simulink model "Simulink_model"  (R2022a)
settings: Solver=VariableStepAuto  StartTime=0.0  StopTime=10.0  RelTol=1e-3
undefined symbols (not defined in the file): Ion, Lithium, sigbuilder_block
libraries: spsMeanLib x15, spsSeriesRLCBranchLib x5, spsIGBTDiodeLib x4, slpidlib x3, spsBatteryLib x2, spsPWMGeneratorDCDCLib x2, spsFirstOrderFilterLib x1, spsCurrentMeasurementLib x1, spsSeriesRLCLoadLib x1, spsVoltageMeasurementLib x1, spspowerguiLib x1

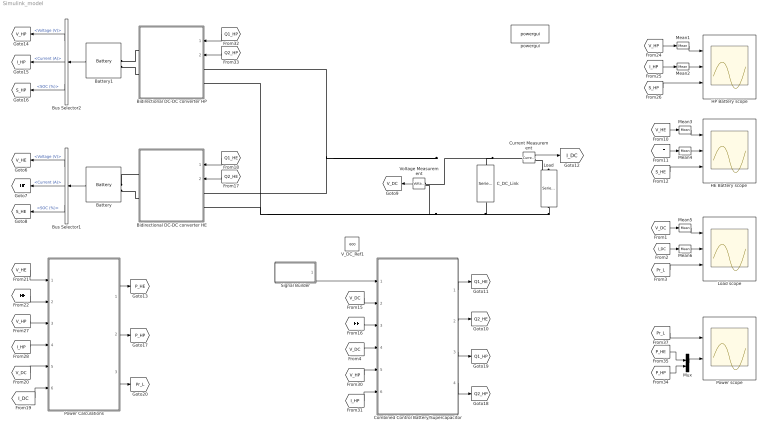
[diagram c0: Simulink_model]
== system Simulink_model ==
  Battery : spsBatteryLib/Battery  BatType=Lithium-Ion  ShowTempParam=off  ThermalPreset=no  ShowAgeParam=off  NomV=300  NomQ=120  SOC=50  Batt_Tr=0.1  PresetModel=on  MaxQ=120  MinV=225  FullV=349.1961  Dis_rate=52.1739  R=0.025  Normal_OP=108.5217  expZone="[324.1158      5.895652]"  current=[6.5 13 32.5]  Units=Time  Tci=20  NomT=20  T2=-30  MaxQ2=4.8  FullV2=7.1  Normal_OP2=5.655  expZone2="[6.58           1]"  Rca=0.6  ti=2000  Dp=0  Neq0=0  Tsim=1e6  Ta1=25  Qeol=5.4*0.9  Reol=0.013333*1.2  Char_age=[2.3478, 3]  Dis_age=[2.3478, 10]  N1=1500  N2=10500  N3=1000  N4=1400  Ta2=45  N5=950
  Battery1 : spsBatteryLib/Battery  BatType=Lithium-Ion  ShowTempParam=off  ThermalPreset=no  ShowAgeParam=off  NomV=100  NomQ=50  SOC=50  Batt_Tr=0.1  PresetModel=on  MaxQ=50  MinV=75  FullV=116.3987  Dis_rate=21.7391  R=0.02  Normal_OP=45.2174  expZone="[108.0386      2.456522]"  current=[6.5 13 32.5]  Units=Time  Tci=20  NomT=20  T2=-30  MaxQ2=4.8  FullV2=7.1  Normal_OP2=5.655  expZone2="[6.58           1]"  Rca=0.6  ti=2000  Dp=0  Neq0=0  Tsim=1e6  Ta1=25  Qeol=5.4*0.9  Reol=0.013333*1.2  Char_age=[2.3478, 3]  Dis_age=[2.3478, 10]  N1=1500  N2=10500  N3=1000  N4=1400  Ta2=45  N5=950
  Bidirectional DC-DC converter HE : Subsystem
  Bidirectional DC-DC converter HP : Subsystem
  Bus Selector1 : BusSelector  OutputSignals=Voltage (V),Current (A),SOC (%)
  Bus Selector2 : BusSelector  OutputSignals=Voltage (V),Current (A),SOC (%)
  C_DC_Link : spsSeriesRLCBranchLib/Series RLC Branch  LConnTagsString=__new0  RConnTagsString=__new0  BranchType=C  Resistance=1  Inductance=1e-3  SetiL0=off  InitialCurrent=0  Capacitance=300e-6  Setx0=off  InitialVoltage=0  Measurements=None
  Combined Control Battery/Supercapacitor : Subsystem
  Current Measurement : spsCurrentMeasurementLib/Current Measurement  PhasorSimulation=off  OutputType=Complex  PSBequivalent=0
  "HE Battery scope " : Scope  NumInputPorts=3
  HP Battery scope : Scope  NumInputPorts=3
  Load : spsSeriesRLCLoadLib/Series RLC Load  LConnTagsString=a  RConnTagsString=__new0  NominalVoltage=50  NominalFrequency=0.00001  ActivePower=500  InductivePower=0  CapacitivePower=0  Setx0=off  InitialVoltage=0  SetiL0=off  InitialCurrent=0  Measurements=None  LoadType=constant Z
  Load scope : Scope  NumInputPorts=3
  Mean{1..6} (6 alike) : spsMeanLib/Mean  Freq=60  Vinit=0  Ts=0
  Mux : Mux  Inputs=2
  Power Calculations : Subsystem
  Power scope : Scope  NumInputPorts=2
  Signal Builder : Subsystem  Tag=STV Subsys  LoadFcn=sigbuilder_block('load');  StartFcn=sigbuilder_block('start');  StopFcn=sigbuilder_block('stop');  ClipboardFcn=sigbuilder_block('clipboard');  mask(Sigbuilder block){tuvar=[0:10]}
      mask help: Simulink:masks:SigbuilderBlock_MD
      mask init:
      | if ~strcmp(get_param(bdroot(gcbh),'SimulationStatus'),'stopped') tuvar = sigbuilder_block('maskInit'); end
  V_DC_Ref1 : Constant  Value=600
  Voltage Measurement : spsVoltageMeasurementLib/Voltage Measurement  PhasorSimulation=off  OutputType=Complex  PSBequivalent=0
  powergui : spspowerguiLib/powergui  Priority=1  SimulationMode=Discrete  SampleTime=1e-6  frequency=60  Iterations=50  frequencyindice=0  Pbase=100e6  ErrMax=1e-4  UnitsV=kV  UnitsW=MW  buscounter=0  FunctionMessages=off  echomessages=off  EnableUseOfTLC=off  CurrentSourceSwitches=off  DisableSnubberDevices=off  DisableRonSwitches=off  DisableVfSwitches=off  DisplayEquations=off  AutomaticDiscreteSolvers=off  SolverType=Tustin/Backward Euler (TBE)  Interpol=off  ExternalGateDelay=off  methode=off  Ts=100  x0status=blocks  SPID=on  SwTol=0  HookPort=off  NonlinearTolerance=1e-4  nMaxIteration=100  ContinueOnMaxIteration=off  RestoreLinks=warning  ResistiveCurrentMeasurement=off  Frange=[0:2:500]  Ylog=off  Xlog=on  ShowGrid=off  save=off  variable=ZData  structure=0  ZoomFFT=off  StartTime=0.0  cycles=1  DisplayStyle=1  fundamental=60  FreqAxis=off  MaxFrequency=1000  frequencyindicesteady=1  RmsSteady=1  display=off
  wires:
  [V_HE] -> Power Calculations/1(V_HE)
  [I_DC] -> Mean6/1
  [V_DC] -> Power Calculations/5(V_DC)
  Bus Selector2/1 -> [V_HP]  "<Voltage (V)>"
  Current Measurement/1 -> [I_DC]
  Bus Selector1/3 -> [S_HE]  "<SOC (%)>"
  [I_HP] -> Mean2/1
  Power Calculations/1(P_HE) -> [P_HE]
  Combined Control Battery/Supercapacitor/1(Q1_HE) -> [Q1_HE]
  Bus Selector2/2 -> [I_HP]  "<Current (A)>"
  [P_HE] -> Mux/1
  [V_DC] -> Combined Control Battery/Supercapacitor/4(V_DC1)
  [P_HP] -> Mux/2
  [Q2_HE] -> Bidirectional DC-DC converter HE/2(D_Q2)
  [Pr_L] -> Load scope/3
  [V_HE] -> Mean3/1
  [V_HP] -> Mean1/1
  [Q1_HE] -> Bidirectional DC-DC converter HE/1(D_Q1)
  Power Calculations/3(P_Load) -> [Pr_L]
  [I_DC] -> Power Calculations/6(I_DC)
  [I_HE] -> Mean4/1
  Combined Control Battery/Supercapacitor/2(Q2_HE) -> [Q2_HE]
  [Q2_HP] -> Bidirectional DC-DC converter HP/2(D_Q2)
  [I_HP] -> Combined Control Battery/Supercapacitor/6(I_HP)
  Bus Selector2/3 -> [S_HP]  "<SOC (%)>"
  [V_HP] -> Power Calculations/3(V_HP)
  [S_HP] -> HP Battery scope/3
  [V_DC] -> Combined Control Battery/Supercapacitor/2(V_DC)
  Battery/1 -> Bus Selector1/1
  [V_DC] -> Mean5/1
  Power Calculations/2(P_HP) -> [P_HP]
  [V_HP] -> Combined Control Battery/Supercapacitor/5("V_HP ")
  Mux/1 -> Power scope/2
  Combined Control Battery/Supercapacitor/4(Q2_HP) -> [Q2_HP]
  Bus Selector1/1 -> [V_HE]  "<Voltage (V)>"
  [I_HP] -> Power Calculations/4(I_HP)
  Combined Control Battery/Supercapacitor/3(Q1_HP) -> [Q1_HP]
  [S_HE] -> "HE Battery scope "/3
  [I_HE] -> Power Calculations/2(I_HE)
  Bus Selector1/2 -> [I_HE]  "<Current (A)>"
  [Q1_HP] -> Bidirectional DC-DC converter HP/1(D_Q1)
  Battery1/1 -> Bus Selector2/1
  [I_HE] -> Combined Control Battery/Supercapacitor/3(I_HE)
  Voltage Measurement/1 -> [V_DC]
  [Pr_L] -> Power scope/1
  Signal Builder/1(Signal 1) -> Combined Control Battery/Supercapacitor/1(VDC_ref)
  Mean1/1 -> HP Battery scope/1
  Mean2/1 -> HP Battery scope/2
  Mean3/1 -> "HE Battery scope "/1
  Mean4/1 -> "HE Battery scope "/2
  Mean5/1 -> Load scope/1
  Mean6/1 -> Load scope/2
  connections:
  Load/RConn1 -- Voltage Measurement/LConn2 -- Bidirectional DC-DC converter HE/LConn2 -- Bidirectional DC-DC converter HP/LConn2 -- C_DC_Link/RConn1
  Current Measurement/LConn1 -- Voltage Measurement/LConn1 -- Bidirectional DC-DC converter HE/LConn1 -- Bidirectional DC-DC converter HP/LConn1 -- C_DC_Link/LConn1
  Bidirectional DC-DC converter HP/RConn1 -- Battery1/LConn1
  Battery/LConn1 -- Bidirectional DC-DC converter HE/RConn1
  Current Measurement/RConn1 -- Load/LConn1
  Bidirectional DC-DC converter HE/RConn2 -- Battery/LConn2
  Bidirectional DC-DC converter HP/RConn2 -- Battery1/LConn2

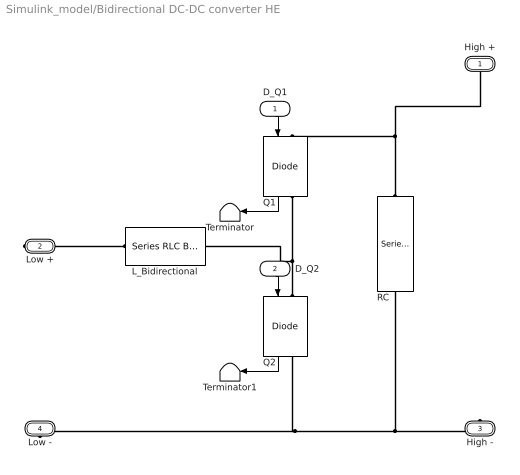
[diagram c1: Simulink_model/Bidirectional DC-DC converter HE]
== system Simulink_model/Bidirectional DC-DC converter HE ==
  D_Q1 : Inport
  D_Q2 : Inport  Port=2
  L_Bidirectional : spsSeriesRLCBranchLib/Series RLC Branch  LConnTagsString=__new0  RConnTagsString=__new0  BranchType=RL  Resistance=0.05  Inductance=0.3e-3  SetiL0=off  InitialCurrent=0  Capacitance=1e-6  Setx0=off  InitialVoltage=0  Measurements=None
  Q1 : spsIGBTDiodeLib/IGBT//Diode  Ron=1e-3  Rs=1e5  Cs=inf  Measurements=on
  Q2 : spsIGBTDiodeLib/IGBT//Diode  Ron=1e-3  Rs=1e5  Cs=inf  Measurements=on
  RC : spsSeriesRLCBranchLib/Series RLC Branch  LConnTagsString=__new0  RConnTagsString=__new0  BranchType=RC  Resistance=0.0001  Inductance=1e-3  SetiL0=off  InitialCurrent=0  Capacitance=1e-6  Setx0=off  InitialVoltage=0  Measurements=None
  Terminator : Terminator
  Terminator1 : Terminator
  High + : PMIOPort  Side=Left
  Low + : PMIOPort  Port=2  Side=Right
  High - : PMIOPort  Port=3  Side=Left
  Low - : PMIOPort  Port=4  Side=Right
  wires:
  Q1/1 -> Terminator/1
  Q2/1 -> Terminator1/1
  D_Q1/1 -> Q1/1
  D_Q2/1 -> Q2/1
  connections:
  Low -/RConn1 -- Q2/RConn1 -- RC/RConn1 -- High -/RConn1
  RC/LConn1 -- Q1/LConn1 -- High +/RConn1
  Low +/RConn1 -- L_Bidirectional/RConn1
  Q2/LConn1 -- Q1/RConn1 -- L_Bidirectional/LConn1

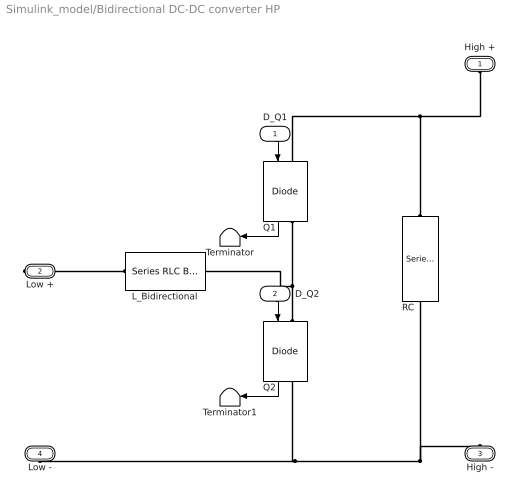
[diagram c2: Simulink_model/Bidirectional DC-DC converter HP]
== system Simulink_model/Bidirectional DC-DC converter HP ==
  D_Q1 : Inport
  D_Q2 : Inport  Port=2
  L_Bidirectional : spsSeriesRLCBranchLib/Series RLC Branch  LConnTagsString=__new0  RConnTagsString=__new0  BranchType=RL  Resistance=0.05  Inductance=.355e-3  SetiL0=off  InitialCurrent=0  Capacitance=1e-6  Setx0=off  InitialVoltage=0  Measurements=None
  Q1 : spsIGBTDiodeLib/IGBT//Diode  Ron=1e-3  Rs=1e5  Cs=inf  Measurements=on
  Q2 : spsIGBTDiodeLib/IGBT//Diode  Ron=1e-3  Rs=1e5  Cs=inf  Measurements=on
  RC : spsSeriesRLCBranchLib/Series RLC Branch  LConnTagsString=__new0  RConnTagsString=__new0  BranchType=RC  Resistance=0.0001  Inductance=1e-3  SetiL0=off  InitialCurrent=0  Capacitance=1e-6  Setx0=off  InitialVoltage=0  Measurements=None
  Terminator : Terminator
  Terminator1 : Terminator
  High + : PMIOPort  Side=Left
  Low + : PMIOPort  Port=2  Side=Right
  High - : PMIOPort  Port=3  Side=Left
  Low - : PMIOPort  Port=4  Side=Right
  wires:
  D_Q2/1 -> Q2/1
  D_Q1/1 -> Q1/1
  Q1/1 -> Terminator/1
  Q2/1 -> Terminator1/1
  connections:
  Low -/RConn1 -- High -/RConn1 -- RC/RConn1 -- Q2/RConn1
  Low +/RConn1 -- L_Bidirectional/RConn1
  Q2/LConn1 -- L_Bidirectional/LConn1 -- Q1/RConn1
  RC/LConn1 -- High +/RConn1 -- Q1/LConn1

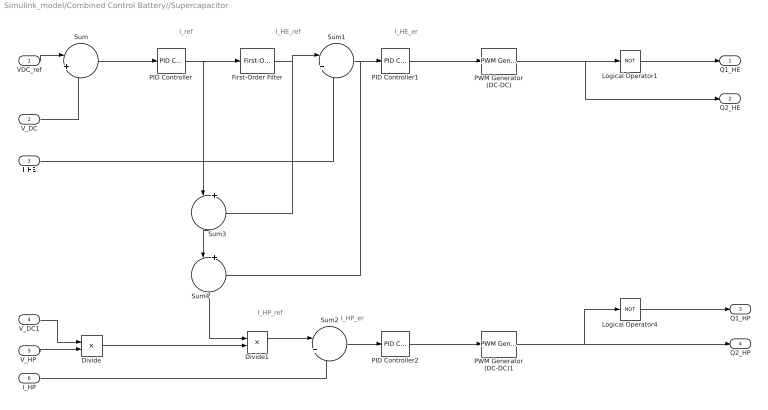
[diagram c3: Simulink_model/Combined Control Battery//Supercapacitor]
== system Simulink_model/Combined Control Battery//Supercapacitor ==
  note: I_HP_er
  note: I_HP_ref
  note: I_HE_er
  note: I_HE_ref
  note: I_ref
  VDC_ref : Inport
  V_DC : Inport  Port=2
  I_HE : Inport  Port=3
  V_DC1 : Inport  Port=4
  "V_HP " : Inport  Port=5
  I_HP : Inport  Port=6
  Divide : Product  Inputs=*/
  Divide1 : Product  Inputs=**
  First-Order Filter : spsFirstOrderFilterLib/First-Order Filter  FilterType=Lowpass  Tc=0.005  Ts=0  Initialize=off  Vac_Init=[0, 0, 60]  Vdc_Init=0  PlotResponse=off  FreqRange="[0,  200,  1]"
  Logical Operator1 : Logic  Operator=NOT  AllPortsSameDT=off  OutDataTypeStr=boolean
  Logical Operator4 : Logic  Operator=NOT  AllPortsSameDT=off  OutDataTypeStr=boolean
  PID Controller : slpidlib/PID Controller  Controller=PI  Form=Parallel  TimeDomain=Continuous-time  UseExternalTs=off  SampleTime=-1  IntegratorMethod=Forward Euler  FilterMethod=Forward Euler  ControllerParametersSource=internal  P=1.477  I=3077  UseKiTs=off  D=0  N=100  UseFilter=on  TunerSelectOption=Transfer Function Based (PID Tuner App)  InitialConditionSource=internal  InitialConditionForIntegrator=0  InitialConditionForFilter=0  DifferentiatorICPrevScaledInput=0  ExternalReset=none  TrackingMode=off  Kt=1  LimitOutput=off  SatLimitsSource=internal  UpperSaturationLimit=inf  LowerSaturationLimit=-inf  LinearizeAsGain=on  AntiWindupMode=none  Kb=1  POutMin=[]  POutMax=[]  IOutMin=[]  IOutMax=[]  DOutMin=[]  DOutMax=[]  NOutMin=[]  NOutMax=[]  SumOutMin=[]  SumOutMax=[]  SaturationOutMin=[]  SaturationOutMax=[]  PParamMin=[]  PParamMax=[]  IParamMin=[]  IParamMax=[]  DParamMin=[]  DParamMax=[]  NParamMin=[]  NParamMax=[]  KbParamMin=[]  KbParamMax=[]  KtParamMin=[]  KtParamMax=[]  KbOutMin=[]  KbOutMax=[]  KtOutMin=[]  KtOutMax=[]  IntegratorOutMin=[]  IntegratorOutMax=[]  FilterOutMin=[]  FilterOutMax=[]  SumI1OutMin=[]  SumI1OutMax=[]  SumI2OutMin=[]  SumI2OutMax=[]  SumI3OutMin=[]  SumI3OutMax=[]  SumI4OutMin=[]  SumI4OutMax=[]  SumDOutMin=[]  SumDOutMax=[]  DifferentiatorOutMin=[]  DifferentiatorOutMax=[]  FilterDiffOutCoefMin=[]  FilterDiffOutCoefMax=[]  ReciprocalOutMin=[]  ReciprocalOutMax=[]  SumDenOutMin=[]  SumDenOutMax=[]  SumNumOutMin=[]  SumNumOutMax=[]  DivideOutMin=[]  DivideOutMax=[]  UdiffTsProdOutMin=[]  UdiffTsProdOutMax=[]  NTsProdOutMin=[]  NTsProdOutMax=[]  UintegralTsProdOutMin=[]  UintegralTsProdOutMax=[]  UngainTsProdOutMin=[]  UngainTsProdOutMax=[]  IntegratorContinuousStateAttributes=''  IntegratorStateMustResolveToSignalObject=off  IntegratorRTWStateStorageClass=Auto  FilterContinuousStateAttributes=''  FilterStateMustResolveToSignalObject=off  FilterRTWStateStorageClass=Auto  ParallelPVariant=InternalParameters  IdealPVariant=Disabled  IVariant=InternalParameters  DVariant=Disabled  IntegratorVariant=Continuous  SatVariant=Disabled  AWVariant=Passthrough  PCopyVariant=Disabled  TRVariant=Disabled  FdbkBlocksVariant=Forward  IdealPFdbkVariant=Disabled  SatFdbkVariant=Disabled  DerivativeFilterVariant=Disabled  NVariant=Disabled  NCopyVariant=Disabled_SignalSpec  FilterICVariant=Disabled  IntegratorICVariant=InternalICs  ExternalResetVariant=Disabled  TRSumVariant=Passthrough  SumFdbkVariant=Disabled  SumVariant=Sum_PI  TsampFilterVariant=InternalTs  TsampNgainVariant=Passthrough  TsampIntegralVariant=Passthrough  ExternalSaturationOutDataTypeStr=Inherit: Same as second input  aMode=0
  PID Controller1 : slpidlib/PID Controller  Controller=PI  Form=Parallel  TimeDomain=Continuous-time  UseExternalTs=off  SampleTime=-1  IntegratorMethod=Forward Euler  FilterMethod=Forward Euler  ControllerParametersSource=internal  P=0.043  I=0.65  UseKiTs=off  D=0  N=100  UseFilter=on  TunerSelectOption=Transfer Function Based (PID Tuner App)  InitialConditionSource=internal  InitialConditionForIntegrator=0  InitialConditionForFilter=0  DifferentiatorICPrevScaledInput=0  ExternalReset=none  TrackingMode=off  Kt=1  LimitOutput=on  SatLimitsSource=internal  UpperSaturationLimit=1  LowerSaturationLimit=0  LinearizeAsGain=on  AntiWindupMode=none  Kb=1  POutMin=[]  POutMax=[]  IOutMin=[]  IOutMax=[]  DOutMin=[]  DOutMax=[]  NOutMin=[]  NOutMax=[]  SumOutMin=[]  SumOutMax=[]  SaturationOutMin=[]  SaturationOutMax=[]  PParamMin=[]  PParamMax=[]  IParamMin=[]  IParamMax=[]  DParamMin=[]  DParamMax=[]  NParamMin=[]  NParamMax=[]  KbParamMin=[]  KbParamMax=[]  KtParamMin=[]  KtParamMax=[]  KbOutMin=[]  KbOutMax=[]  KtOutMin=[]  KtOutMax=[]  IntegratorOutMin=[]  IntegratorOutMax=[]  FilterOutMin=[]  FilterOutMax=[]  SumI1OutMin=[]  SumI1OutMax=[]  SumI2OutMin=[]  SumI2OutMax=[]  SumI3OutMin=[]  SumI3OutMax=[]  SumI4OutMin=[]  SumI4OutMax=[]  SumDOutMin=[]  SumDOutMax=[]  DifferentiatorOutMin=[]  DifferentiatorOutMax=[]  FilterDiffOutCoefMin=[]  FilterDiffOutCoefMax=[]  ReciprocalOutMin=[]  ReciprocalOutMax=[]  SumDenOutMin=[]  SumDenOutMax=[]  SumNumOutMin=[]  SumNumOutMax=[]  DivideOutMin=[]  DivideOutMax=[]  UdiffTsProdOutMin=[]  UdiffTsProdOutMax=[]  NTsProdOutMin=[]  NTsProdOutMax=[]  UintegralTsProdOutMin=[]  UintegralTsProdOutMax=[]  UngainTsProdOutMin=[]  UngainTsProdOutMax=[]  IntegratorContinuousStateAttributes=''  IntegratorStateMustResolveToSignalObject=off  IntegratorRTWStateStorageClass=Auto  FilterContinuousStateAttributes=''  FilterStateMustResolveToSignalObject=off  FilterRTWStateStorageClass=Auto  ParallelPVariant=InternalParameters  IdealPVariant=Disabled  IVariant=InternalParameters  DVariant=Disabled  IntegratorVariant=Continuous  SatVariant=Enabled  AWVariant=Passthrough  PCopyVariant=Disabled  TRVariant=Disabled  FdbkBlocksVariant=Forward  IdealPFdbkVariant=Disabled  SatFdbkVariant=Disabled  DerivativeFilterVariant=Disabled  NVariant=Disabled  NCopyVariant=Disabled_SignalSpec  FilterICVariant=Disabled  IntegratorICVariant=InternalICs  ExternalResetVariant=Disabled  TRSumVariant=Passthrough  SumFdbkVariant=Disabled  SumVariant=Sum_PI  TsampFilterVariant=InternalTs  TsampNgainVariant=Passthrough  TsampIntegralVariant=Passthrough  ExternalSaturationOutDataTypeStr=Inherit: Same as second input  aMode=0
  PID Controller2 : slpidlib/PID Controller  Controller=PI  Form=Parallel  TimeDomain=Continuous-time  UseExternalTs=off  SampleTime=-1  IntegratorMethod=Forward Euler  FilterMethod=Forward Euler  ControllerParametersSource=internal  P=0.043  I=0.65  UseKiTs=off  D=0  N=100  UseFilter=on  TunerSelectOption=Transfer Function Based (PID Tuner App)  InitialConditionSource=internal  InitialConditionForIntegrator=0  InitialConditionForFilter=0  DifferentiatorICPrevScaledInput=0  ExternalReset=none  TrackingMode=off  Kt=1  LimitOutput=on  SatLimitsSource=internal  UpperSaturationLimit=1  LowerSaturationLimit=0  LinearizeAsGain=on  AntiWindupMode=none  Kb=1  POutMin=[]  POutMax=[]  IOutMin=[]  IOutMax=[]  DOutMin=[]  DOutMax=[]  NOutMin=[]  NOutMax=[]  SumOutMin=[]  SumOutMax=[]  SaturationOutMin=[]  SaturationOutMax=[]  PParamMin=[]  PParamMax=[]  IParamMin=[]  IParamMax=[]  DParamMin=[]  DParamMax=[]  NParamMin=[]  NParamMax=[]  KbParamMin=[]  KbParamMax=[]  KtParamMin=[]  KtParamMax=[]  KbOutMin=[]  KbOutMax=[]  KtOutMin=[]  KtOutMax=[]  IntegratorOutMin=[]  IntegratorOutMax=[]  FilterOutMin=[]  FilterOutMax=[]  SumI1OutMin=[]  SumI1OutMax=[]  SumI2OutMin=[]  SumI2OutMax=[]  SumI3OutMin=[]  SumI3OutMax=[]  SumI4OutMin=[]  SumI4OutMax=[]  SumDOutMin=[]  SumDOutMax=[]  DifferentiatorOutMin=[]  DifferentiatorOutMax=[]  FilterDiffOutCoefMin=[]  FilterDiffOutCoefMax=[]  ReciprocalOutMin=[]  ReciprocalOutMax=[]  SumDenOutMin=[]  SumDenOutMax=[]  SumNumOutMin=[]  SumNumOutMax=[]  DivideOutMin=[]  DivideOutMax=[]  UdiffTsProdOutMin=[]  UdiffTsProdOutMax=[]  NTsProdOutMin=[]  NTsProdOutMax=[]  UintegralTsProdOutMin=[]  UintegralTsProdOutMax=[]  UngainTsProdOutMin=[]  UngainTsProdOutMax=[]  IntegratorContinuousStateAttributes=''  IntegratorStateMustResolveToSignalObject=off  IntegratorRTWStateStorageClass=Auto  FilterContinuousStateAttributes=''  FilterStateMustResolveToSignalObject=off  FilterRTWStateStorageClass=Auto  ParallelPVariant=InternalParameters  IdealPVariant=Disabled  IVariant=InternalParameters  DVariant=Disabled  IntegratorVariant=Continuous  SatVariant=Enabled  AWVariant=Passthrough  PCopyVariant=Disabled  TRVariant=Disabled  FdbkBlocksVariant=Forward  IdealPFdbkVariant=Disabled  SatFdbkVariant=Disabled  DerivativeFilterVariant=Disabled  NVariant=Disabled  NCopyVariant=Disabled_SignalSpec  FilterICVariant=Disabled  IntegratorICVariant=InternalICs  ExternalResetVariant=Disabled  TRSumVariant=Passthrough  SumFdbkVariant=Disabled  SumVariant=Sum_PI  TsampFilterVariant=InternalTs  TsampNgainVariant=Passthrough  TsampIntegralVariant=Passthrough  ExternalSaturationOutDataTypeStr=Inherit: Same as second input  aMode=0
  PWM Generator (DC-DC) : spsPWMGeneratorDCDCLib/PWM Generator (DC-DC)  Fsw=16000  Ts=0
  PWM Generator (DC-DC)1 : spsPWMGeneratorDCDCLib/PWM Generator (DC-DC)  Fsw=16000  Ts=0
  Sum{,1..3} (4 alike) : Sum  Inputs=|+-
  Sum4 : Sum  Inputs=|++
  Q1_HE : Outport
  Q2_HE : Outport  Port=2
  Q1_HP : Outport  Port=3
  Q2_HP : Outport  Port=4
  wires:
  Sum1/1 -> PID Controller1/1, Sum4/2
  PWM Generator (DC-DC)/1 -> Logical Operator1/1, Q2_HE/1
  I_HE/1 -> Sum1/2
  I_HP/1 -> Sum2/2
  Sum2/1 -> PID Controller2/1
  Sum/1 -> PID Controller/1
  VDC_ref/1 -> Sum/1
  V_DC/1 -> Sum/2
  V_DC1/1 -> Divide/1
  "V_HP "/1 -> Divide/2
  Sum3/1 -> Sum4/1
  Divide1/1 -> Sum2/1
  Divide/1 -> Divide1/2
  Sum4/1 -> Divide1/1
  PID Controller2/1 -> PWM Generator (DC-DC)1/1
  PID Controller1/1 -> PWM Generator (DC-DC)/1
  First-Order Filter/1 -> Sum1/1, Sum3/2
  PWM Generator (DC-DC)1/1 -> Q2_HP/1, Logical Operator4/1
  PID Controller/1 -> First-Order Filter/1, Sum3/1
  Logical Operator1/1 -> Q1_HE/1
  Logical Operator4/1 -> Q1_HP/1

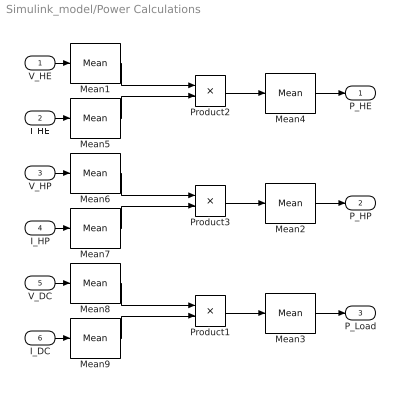
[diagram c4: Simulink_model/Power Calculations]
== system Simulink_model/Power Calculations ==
  V_HE : Inport
  I_HE : Inport  Port=2
  V_HP : Inport  Port=3
  I_HP : Inport  Port=4
  V_DC : Inport  Port=5
  I_DC : Inport  Port=6
  Mean{1..9} (9 alike) : spsMeanLib/Mean  Freq=60  Vinit=0  Ts=0
  Product1 : Product
  Product2 : Product
  Product3 : Product
  P_HE : Outport
  P_HP : Outport  Port=2
  P_Load : Outport  Port=3
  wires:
  I_HE/1 -> Mean5/1
  V_HE/1 -> Mean1/1
  V_DC/1 -> Mean8/1
  I_DC/1 -> Mean9/1
  V_HP/1 -> Mean6/1
  I_HP/1 -> Mean7/1
  Mean4/1 -> P_HE/1
  Product2/1 -> Mean4/1
  Mean2/1 -> P_HP/1
  Product3/1 -> Mean2/1
  Mean3/1 -> P_Load/1
  Product1/1 -> Mean3/1
  Mean1/1 -> Product2/1
  Mean5/1 -> Product2/2
  Mean6/1 -> Product3/1
  Mean7/1 -> Product3/2
  Mean8/1 -> Product1/1
  Mean9/1 -> Product1/2

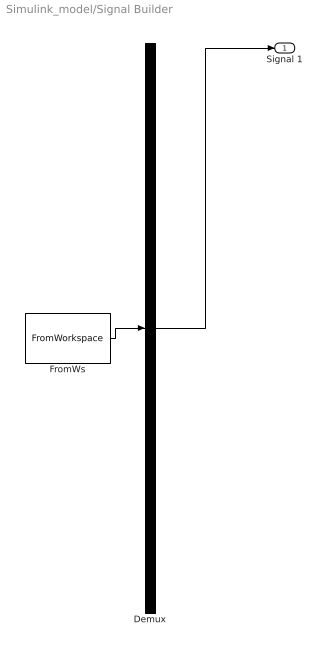
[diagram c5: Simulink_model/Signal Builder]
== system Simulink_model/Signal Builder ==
  Demux : Demux  Tag=STV Demux  Outputs=1
  FromWs : FromWorkspace  Tag=STV FromWs  VariableName=tuvar
  Signal 1 : Outport  Tag=STV Outport
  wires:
  Demux/1 -> Signal 1/1
  FromWs/1 -> Demux/1
